(* Logix 5000 Rung export; software revision 19.01 *)

TYPE PLX51DF1MSGOutput :
STRUCT
   RoutingInhibit : BOOL;
END_STRUCT
END_TYPE

TYPE PLX51DF1MSGDataType :
STRUCT
   BOOLEAN : BOOL;
   INT : BOOL;
   REAL : BOOL;
END_STRUCT
END_TYPE

TYPE PLX51DF1MSGInput :
STRUCT
   Instance : STRING;
   Status : PLX51DF1MSGStatus;
   TransactionRate : DINT;
   Temperature : REAL;
   DF1RxPacketCount : DINT;
   DF1TxPacketCount : DINT;
   DF1ChecksumErrors : DINT;
   PCCCRequests : DINT;
   PCCCFailures : DINT;
   TagReads : DINT;
   TagWrites : DINT;
   TagConnectionFailures : DINT;
   TagErrors : DINT;
END_STRUCT
END_TYPE

TYPE PLX51DF1MSGStatus :
STRUCT
   Reserved0 : BOOL;
   DF1SlaveMode : BOOL;
   ScheduledMode : BOOL;
   Reserved1 : BOOL;
   ConfigurationValid : BOOL;
   RoutingInhibited : BOOL;
   Reserved3 : BOOL;
   Reserved4 : BOOL;
   ScheduledTagStatus0 : BOOL;
   ScheduledTagStatus1 : BOOL;
   ScheduledTagStatus2 : BOOL;
   ScheduledTagStatus3 : BOOL;
   ScheduledTagStatus4 : BOOL;
   ScheduledTagStatus5 : BOOL;
   ScheduledTagStatus6 : BOOL;
   ScheduledTagStatus7 : BOOL;
   ScheduledTagStatus8 : BOOL;
   ScheduledTagStatus9 : BOOL;
   ScheduledTagStatus10 : BOOL;
   ScheduledTagStatus11 : BOOL;
   ScheduledTagStatus12 : BOOL;
   ScheduledTagStatus13 : BOOL;
   ScheduledTagStatus14 : BOOL;
   ScheduledTagStatus15 : BOOL;
   ScheduledTagStatus16 : BOOL;
   ScheduledTagStatus17 : BOOL;
   ScheduledTagStatus18 : BOOL;
   ScheduledTagStatus19 : BOOL;
END_STRUCT
END_TYPE

TYPE PLX51MessengerMsgResponse :
STRUCT
   Status : INT;
   ResponseLength : INT;
   ResponseData : INT[128];
END_STRUCT
END_TYPE

TYPE PLX51MessengerMsgRequest :
STRUCT
   DestinationNode : INT;
   DF1DataFileAddress : STRING;
   Function : PLX51DF1MSGFunctionType;
   DataType : PLX51DF1MSGDataType;
   ElementCount : INT;
   RequestData : INT[128];
END_STRUCT
END_TYPE

TYPE PLX51DF1MSGFunctionType :
STRUCT
   PLC5TypedRead : BOOL;
   PLC5TypedWrite : BOOL;
   SLCTypedRead : BOOL;
   SLCTypedWrite : BOOL;
END_STRUCT
END_TYPE

VAR_GLOBAL   (* controller tags *)
   DF1MSGMsgResponse : PLX51MessengerMsgResponse;
   DF1MSGInput : PLX51DF1MSGInput := (Instance := 'DF1 Messenger', Status.DF1SlaveMode := 1, Status.ConfigurationValid := 1);
   DF1Messenger:O : AB:ETHERNET_MODULE_DINT_4Bytes:O:0;
   DF1MSGMsgRequest : PLX51MessengerMsgRequest := (DestinationNode := 5, DF1DataFileAddress := 'N10:0', Function.PLC5TypedRead := 1, DataType.INT := 1, ElementCount := 16);
   DF1MsgTrigger : BOOL;
   DF1MSGMessage : MESSAGE;
        MessageParameters(MessageType := CIP Generic, RequestedLength := 360, ConnectedFlag := 2, ConnectionPath := DF1Messenger, ServiceCode := 16#006a, ObjectType := 16#0408, TargetObject := 1, LocalElement := DF1MSGMsgRequest, DestinationTag := DF1MSGMsgResponse)
   DF1Messenger:I : AB:ETHERNET_MODULE_DINT_136Bytes:I:0 := (Data[0] := 9, Data[1] := 1378960964, Data[2] := 1702131055, Data[3] := 114, Data[22] := 6, Data[23] := 31, Data[24] := 1111061090, Data[25] := 318107, Data[26] := 318184, Data[30] := 82158, Data[31] := 76934);
   DF1MSGOutput : PLX51DF1MSGOutput;
END_VAR

PROGRAM MainProgram

ROUTINE MainRoutine   (* ladder *)
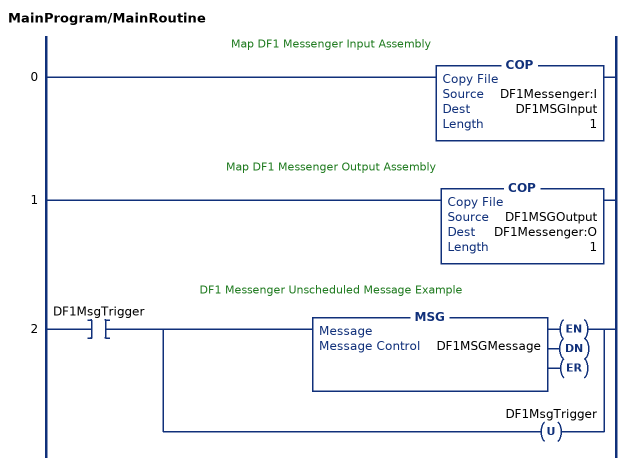
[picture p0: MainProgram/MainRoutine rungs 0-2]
   // Map DF1 Messenger Input Assembly
   0: COP(DF1Messenger:I,DF1MSGInput,1);
   // Map DF1 Messenger Output Assembly
   1: COP(DF1MSGOutput,DF1Messenger:O,1);
   // DF1 Messenger Unscheduled Message Example
   2: XIC(DF1MsgTrigger)[MSG(DF1MSGMessage) ,OTU(DF1MsgTrigger) ];
END_ROUTINE
END_PROGRAM
